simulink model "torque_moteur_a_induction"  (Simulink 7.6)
settings: Solver=ode15s  StartTime=0.0  StopTime=20.0  RelTol=1e-3
InitFcn:
  | % valeurs des composants électriques
  | R1=1;
  | R2=1;
  | L1=0.02;
  | L2=0.02;
  | Lm=0.5;
  | n=3;
  | p=1;
  | 
  | % signal d'alimentation des phases du stator
  | Vrms=220/sqrt(2);
  | f=60;
StopFcn:
  | close all
  | load torque_mot_inductiont.mat
  | plotyy(x(1,:),x(2,:),x(1,:),x(3,:))
  | title('Position et Vitesse du rotor')
  | xlabel('temps')
  | grid
  | 
  | figure
  | 
  | plot (x(1,:),x(4,:))
  | %axis([5.8 6.4 1 3.5])
  | grid
  | title('Couple sur l''arbre moteur')
  | xlabel('temps')
libraries: fl_lib x6, nesl_utility x6, elec_lib x1

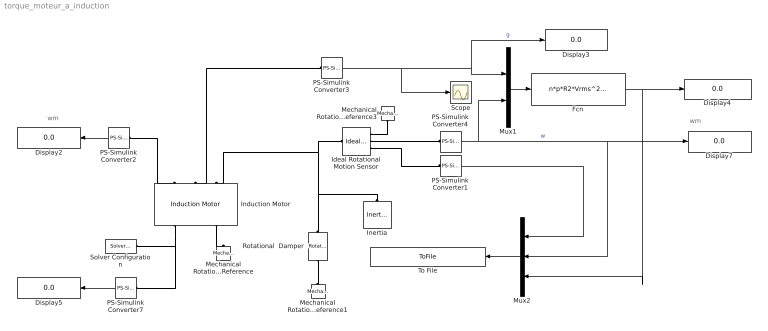
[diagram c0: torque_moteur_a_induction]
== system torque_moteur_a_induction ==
  note: wm
  note: wm
  Display{2..5,7} (5 alike) : Display
  Fcn : Fcn  Expr=n*p*R2*Vrms^2/(u(1)*u(2))/((R1+R2+(1-u(1))*R2/u(1))^2+(1/(L1*2*pi*f)+1/(L2*2*pi*f))^2)
  Ideal Rotational Motion Sensor : fl_lib/Mechanical/Mechanical Sensors/Ideal Rotational Motion Sensor  DialogController=NetworkEngine.DynNeDlgSource  SystemSampleTime=-1  offset=0 rad  w_Log=off  t_Log=off  phi_Log=off  LocalVarNames=|w|t|phi  LocalVarDescs=|w|t|phi  LocalVarLogging=[0 0 0]
  Induction Motor : elec_lib/Actuators & Drivers/Rotational Actuators/Induction Motor  DialogController=NetworkEngine.DynNeDlgSource  SystemSampleTime=-1  param=2  R1=R1 Ohm  R2=R2 Ohm  L1=L1 H  L2=L2 H  Lm=Lm H  P_rated=825 W  w_mech=3.5e+03 rpm  v_rated=200 V  w_rated=60 Hz  i_rated=2.7 A  paramL=1  i_start=7.5 A  T_max=3.3 N*m  paramR1=1  E=95  pf=0.93  R1m=1 Ohm  V=Vrms V  w=f Hz  p=p  n=n  paramLoad=1  J=0.001 kg*m^2  lam=1e-04 N*m/(rad/s)  speed0=0 rpm  LocalVarLogging=[]
  Inertia : fl_lib/Mechanical/Rotational Elements/Inertia  DialogController=NetworkEngine.DynNeDlgSource  SystemSampleTime=-1  inertia=0.01 kg*m^2  initial_velocity=0 rad/s  t_Log=off  LocalVarNames=|t  LocalVarDescs=|t  LocalVarLogging=0
  Mechanical Rotational Reference : fl_lib/Mechanical/Rotational Elements/Mechanical Rotational Reference  DialogController=NetworkEngine.DynNeDlgSource  SystemSampleTime=-1  t_Log=off  LocalVarNames=|t  LocalVarDescs=|t  LocalVarLogging=0
  Mechanical Rotational Reference1 : fl_lib/Mechanical/Rotational Elements/Mechanical Rotational Reference  DialogController=NetworkEngine.DynNeDlgSource  SystemSampleTime=-1  t_Log=off  LocalVarNames=|t  LocalVarDescs=|t  LocalVarLogging=0
  Mechanical Rotational Reference3 : fl_lib/Mechanical/Rotational Elements/Mechanical Rotational Reference  DialogController=NetworkEngine.DynNeDlgSource  SystemSampleTime=-1  t_Log=off  LocalVarNames=|t  LocalVarDescs=|t  LocalVarLogging=0
  Mux1 : Mux  Inputs=2
  Mux2 : Mux  Inputs=3
  PS-Simulink Converter1 : nesl_utility/PS-Simulink Converter  DialogController=NetworkEngine.DynNeUtilDlgSource  SystemSampleTime=-1  PhysicalDomain=network_engine_domain  LeftPortType=input  RightPortType=output  SubClassName=ps_output  Unit=rad  AffineConversion=off
  PS-Simulink Converter2 : nesl_utility/PS-Simulink Converter  DialogController=NetworkEngine.DynNeUtilDlgSource  SystemSampleTime=-1  PhysicalDomain=network_engine_domain  LeftPortType=input  RightPortType=output  SubClassName=ps_output  Unit=1  AffineConversion=off
  PS-Simulink Converter3 : nesl_utility/PS-Simulink Converter  DialogController=NetworkEngine.DynNeUtilDlgSource  SystemSampleTime=-1  PhysicalDomain=network_engine_domain  LeftPortType=input  RightPortType=output  SubClassName=ps_output  Unit=1  AffineConversion=off
  PS-Simulink Converter4 : nesl_utility/PS-Simulink Converter  DialogController=NetworkEngine.DynNeUtilDlgSource  SystemSampleTime=-1  PhysicalDomain=network_engine_domain  LeftPortType=input  RightPortType=output  SubClassName=ps_output  Unit=rad/s  AffineConversion=off
  PS-Simulink Converter7 : nesl_utility/PS-Simulink Converter  DialogController=NetworkEngine.DynNeUtilDlgSource  SystemSampleTime=-1  PhysicalDomain=network_engine_domain  LeftPortType=input  RightPortType=output  SubClassName=ps_output  Unit=W  AffineConversion=off
  Rotational  Damper : fl_lib/Mechanical/Rotational Elements/Rotational Damper  DialogController=NetworkEngine.DynNeDlgSource  SystemSampleTime=-1  D=0.001 N*m/(rad/s)  t_Log=off  w_Log=off  LocalVarNames=|t|w  LocalVarDescs=|t|w  LocalVarLogging=[0 0]
  Scope : Scope
  Solver Configuration : nesl_utility/Solver Configuration  DialogController=NetworkEngine.DynNeUtilDlgSource  SystemSampleTime=-1  PhysicalDomain=network_engine_domain  LeftPortType=input  RightPortType=generic  SubClassName=solver  Accelerate=off  Profile=off  ResidualTolerance=1e-9  MaxNonlinIter=12  MaxModeIter=2  DoFixedCost=off  UseLocalSampling=off  DoDC=off  LinearAlgebra=Sparse  LocalSolverSampleTime=.001  LocalSolverChoice=NE_BACKWARD_EULER_ADVANCER  UseLocalSolver=off
  To File : ToFile  Filename=torque_mot_inductiont.mat  MatrixName=x
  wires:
  PS-Simulink Converter2/1 -> Display2/1
  Mux1/1 -> Fcn/1
  PS-Simulink Converter4/1 -> Mux1/2, Display7/1, Mux2/2  "w"
  Fcn/1 -> Display4/1, Mux2/3
  PS-Simulink Converter3/1 -> Mux1/1, Display3/1, Scope/1  "g"
  PS-Simulink Converter7/1 -> Display5/1
  Mux2/1 -> To File/1
  PS-Simulink Converter1/1 -> Mux2/1
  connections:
  Induction Motor/RConn1 -- Solver Configuration/RConn1 -- PS-Simulink Converter7/LConn1
  PS-Simulink Converter2/LConn1 -- Induction Motor/LConn1
  Induction Motor/RConn3 -- Mechanical Rotational Reference/LConn1
  Inertia/LConn1 -- Ideal Rotational Motion Sensor/LConn1 -- Induction Motor/LConn3 -- Rotational  Damper/LConn1
  Rotational  Damper/RConn1 -- Mechanical Rotational Reference1/LConn1
  Mechanical Rotational Reference3/LConn1 -- Ideal Rotational Motion Sensor/RConn1
  Ideal Rotational Motion Sensor/RConn2 -- PS-Simulink Converter4/LConn1
  PS-Simulink Converter3/LConn1 -- Induction Motor/LConn2
  Ideal Rotational Motion Sensor/RConn3 -- PS-Simulink Converter1/LConn1
